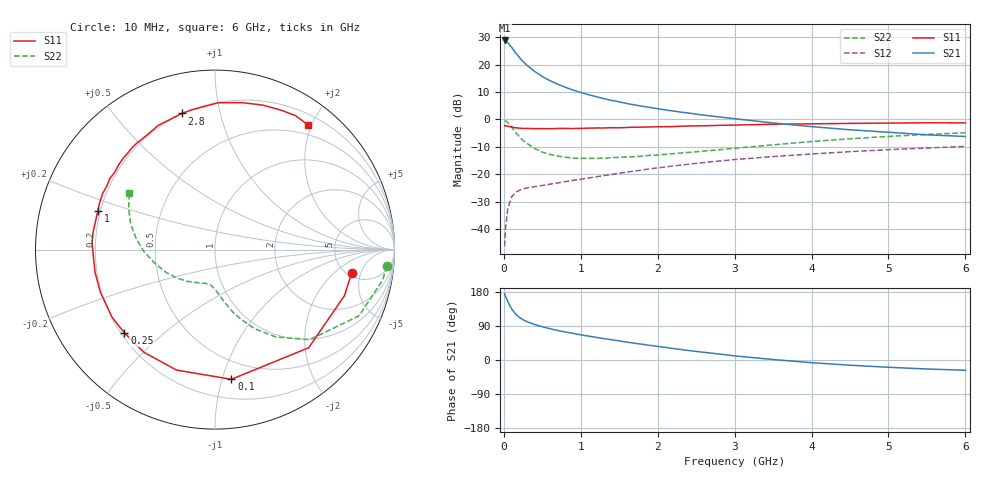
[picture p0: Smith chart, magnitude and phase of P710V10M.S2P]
! SIEMENS Small Signal Semiconductors
! BFP196
! Si NPN RF Bipolar Junction Transistor in SOT143
! VCE = 10 V  IC = 10 mA
! Common Emitter S-Parameters:  May  1996
# GHz  S  MA  R  50
!  f  S11  S21  S12  S22
! GHz  MAG  ANG  MAG  ANG  MAG  ANG  MAG  ANG
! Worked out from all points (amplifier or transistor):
!   36 points, 10 MHz to 6 GHz, reference 50 ohm
!   highest |S21| = 28.8 dB at 10 MHz (marker M1)
!   |S21| within 3 dB of that: start of sweep to 113.7 MHz
!   unconditionally stable (mu >= 1): 931.2 MHz to 3.363 GHz
!   at 250 MHz: K = 0.39, MSG = 23.2 dB, |S12| = -25.3 dB
!   at 1.4 GHz: K = 1.12, MAG = 11.4 dB, |S12| = -20.1 dB
!   at 6 GHz: K = 0.96, MSG = 1.8 dB, |S12| = -9.8 dB
!   S11 on the Smith chart (normalised r, x): 10 MHz: 5.42, -3.53; 100 MHz: 0.35, -1.07; 250 MHz: 0.21, -0.37; 1 GHz: 0.19, +0.16; 2.8 GHz: 0.20, +0.77; 6 GHz: 0.35, +1.94
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0.01  0.7721 -9.8  27.57 175.3  0.0049 83.8  0.9623 -5.5
0.02  0.7656 -19.6  26.79 169.0  0.0098 77.6  0.9491 -10.4
0.05  0.756 -46.3  25.17 154.6  0.0232 67.6  0.883 -24.7
0.1  0.7284 -82.8  20.76 135.4  0.0385 53.2  0.7286 -43.5
0.15  0.7046 -107.7  16.57 121.8  0.0466 43.2  0.5912 -55.3
0.2  0.6959 -124.8  13.66 112.8  0.051 38.4  0.4891 -63.7
0.25  0.6855 -137.4  11.35 106.0  0.0542 35.0  0.4143 -69.5
0.3  0.6864 -146.6  9.726 101.2  0.0565 33.6  0.3666 -73.7
0.4  0.6813 -159.8  7.531 93.7  0.0596 32.6  0.2954 -80.0
0.5  0.6801 -169.2  6.067 87.8  0.0627 33.3  0.2539 -84.6
0.6  0.6788 -176.7  5.096 82.6  0.0662 34.4  0.2303 -88.2
0.7  0.6864 176.5  4.405 77.9  0.0695 35.8  0.2157 -91.5
0.8  0.6858 171.4  3.861 73.9  0.0736 36.9  0.205 -94.7
1  0.6878 161.6  3.105 66.5  0.0811 39.4  0.1956 -100.3
1.1  0.6946 157.5  2.835 63.0  0.0856 40.3  0.1952 -103.0
1.6  0.7147 138.8  1.953 47.2  0.1098 42.5  0.2076 -116.4
2.2  0.7426 120.4  1.425 30.4  0.1419 41.2  0.2382 -132.1
2.8  0.7808 103.7  1.111 15.7  0.1747 37.0  0.2802 -149.4
3.5  0.8185 88.7  0.863 1.3  0.2108 30.2  0.3443 -167.3
4.5  0.848 71.6  0.649 -13.8  0.259 19.9  0.4447 171.7
5.5  0.8711 59.0  0.525 -23.7  0.3022 8.9  0.5339 154.4
6  0.8667 53.4  0.49 -27.1  0.3223 2.8  0.5716 146.5
